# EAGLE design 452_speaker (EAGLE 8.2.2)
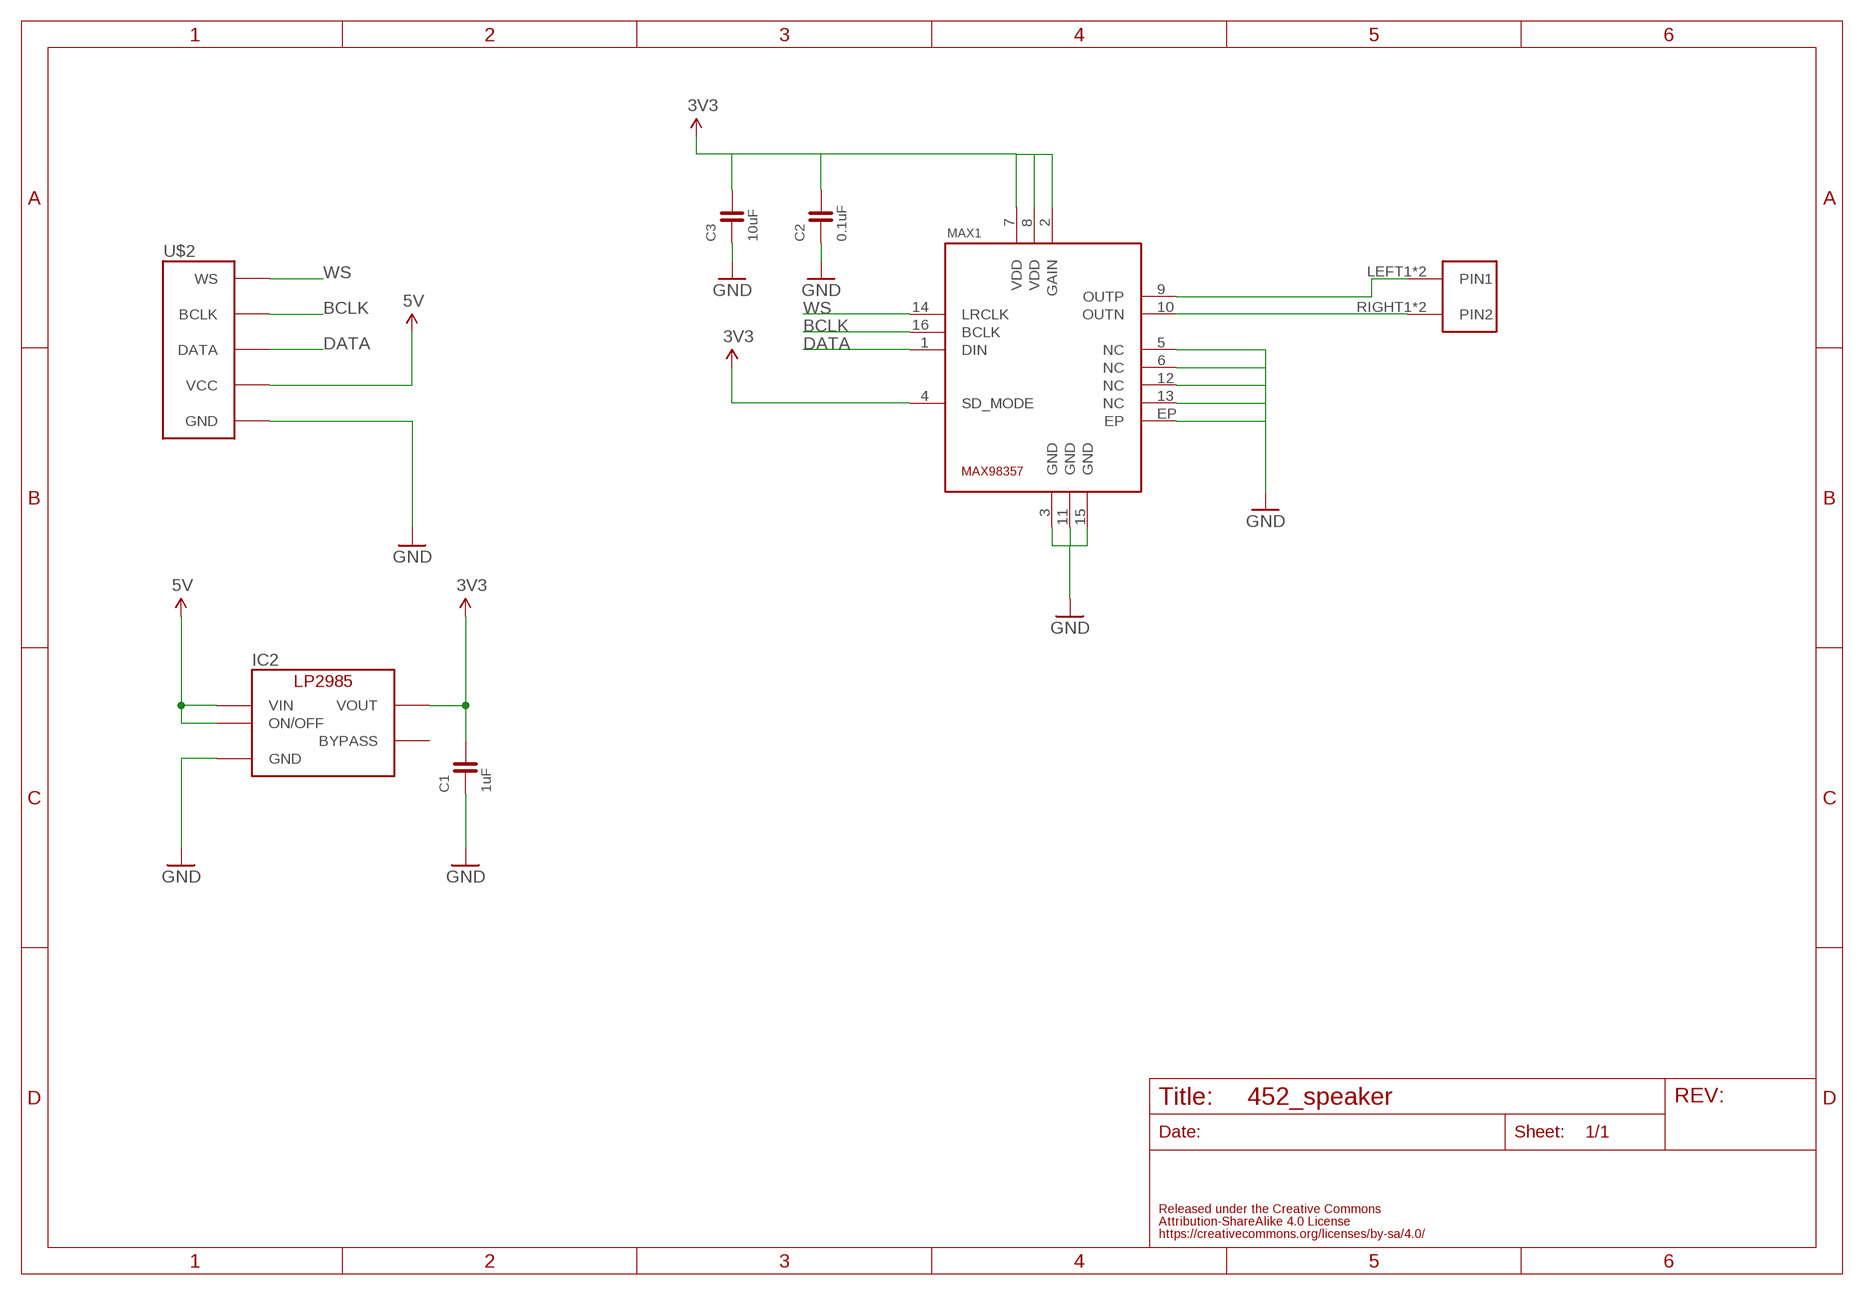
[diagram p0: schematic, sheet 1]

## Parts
C1  1uF  CAPACITOR-0603  [0603]
C2  0.1uF  CAPACITOR-0603  [0603]
C3  10uF  CAPACITOR-0603  [0603]
IC2  LP2985-33DBV  [SOT-23-5]
MAX1  MA-MAX98357  [MAXIM-MAX98357]
U$2  FABO_BRICK_I2S  [FABO_BRICK_I2S]
U$4  ML-1400-S1  [ML-1400-S1]

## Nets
3V3: C1.2 C2.2 C3.2 IC2.5(VOUT) MAX1.2(GAIN) MAX1.4(SD_MODE) MAX1.7(VDD) MAX1.8(VDD)
5V: IC2.1(VIN) IC2.3(ON/OFF) U$2.VCC
BCLK: MAX1.16(BCLK) U$2.BCLK
DATA: MAX1.1(DIN) U$2.DATA
GND: C1.1 C2.1 C3.1 IC2.2(GND) MAX1.3(GND) MAX1.5(NC) MAX1.6(NC) MAX1.11(GND) MAX1.12(NC) MAX1.13(NC) MAX1.15(GND) MAX1.EP U$2.GND
N$1: MAX1.10(OUTN) U$4.RIGHT1(PIN2) U$4.RIGHT2(PIN2)
N$2: MAX1.9(OUTP) U$4.LEFT1(PIN1) U$4.LEFT2(PIN1)
WS: MAX1.14(LRCLK) U$2.WS
Unconnected: IC2.4(BYPASS)

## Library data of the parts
C1-C3 = FaBo-Capacitor:CAPACITOR: CAPACITOR
IC2 = FaBo-Supply:LP2985: LP2985
MAX1 = FaBo-Mems:MA-MAX98357
U$2 = FaBo-Template:FABO_BRICK_I2S
U$4 = FaBo-Terminal:ML-1400-S1

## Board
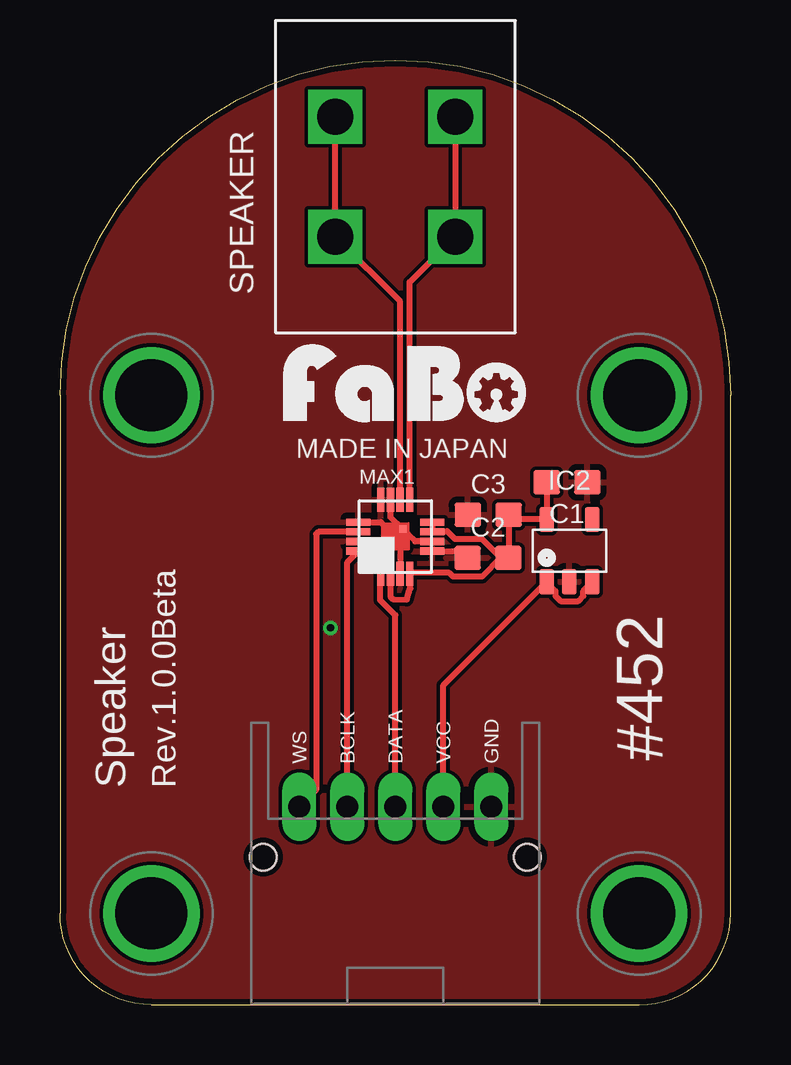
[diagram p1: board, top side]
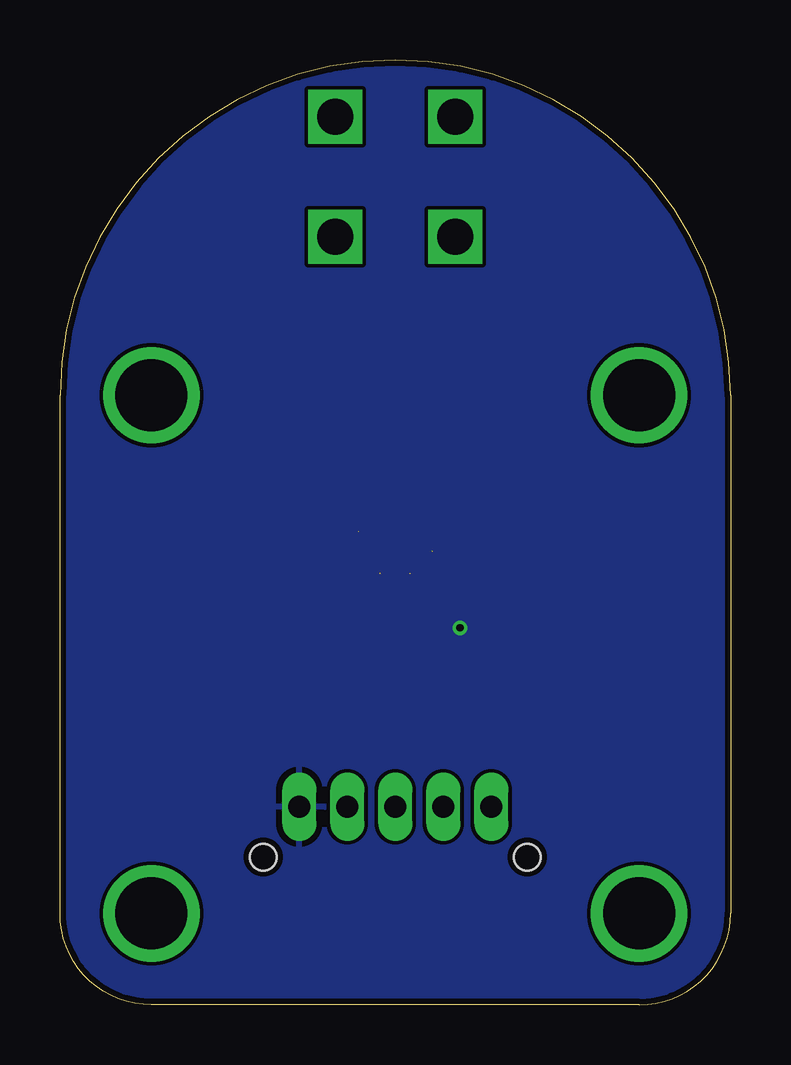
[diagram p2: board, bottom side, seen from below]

Size 27.94 x 39.37 mm. Coordinates in mm from the lower left corner, seen from the top.
Copper layers (1*16): Top 0.035mm / dielectric 1.5mm / Bottom 0.035mm
Design rules "Elecrow_angle": minimum track width 6mil, minimum drill 12mil, track to track 6mil, track to pad 6mil, pad to pad 6mil, via to via 6mil, smd to smd 0mil, copper to edge 10mil, drill to drill 10mil, minimum pad ring 10mil, minimum via ring 6mil, stop-mask expansion 2mil, vias tented up to drill 100mil, thermal gap 10mil

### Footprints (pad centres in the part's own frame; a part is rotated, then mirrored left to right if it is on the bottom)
0603 = smd 1.1 x 1: 1 -0.85,0; 2 0.85,0
SOT-23-5 = smd 0.6 x 1.05: 1 -0.95,-1.3; 2 0,-1.3; 3 0.95,-1.3; 4 0.95,1.3; 5 -0.95,1.3
MAXIM-MAX98357 = smd 0.3 x 1: 1 -0.6,-1.54; 2 -0.2,-1.54; 3 0.2,-1.54; 4 0.6,-1.54; 9 0.6,1.54; 10 0.2,1.54; 11 -0.2,1.54; 12 -0.6,1.54 | smd 1 x 0.3: 5 1.54,-0.6; 6 1.54,-0.2; 7 1.54,0.2; 8 1.54,0.6; 13 -1.54,0.6; 14 -1.54,0.2; 15 -1.54,-0.2; 16 -1.54,-0.6 | smd 0.3 x 0.3: EP 0.31,0.32
FABO_BRICK_I2S = drill 0.9 pad 1.422 long: BCLK -2,-8.255; DATA 0,-8.255; GND 4,-8.255; VCC 2,-8.255; WS -4,-8.255 | drill 3 pad 3.81: P$1 -10.16,8.89; P$2 10.16,8.89; P$3 -10.16,-12.7; P$4 10.16,-12.7 | hole 1.1: -5.5,-10.355; 5.5,-10.355
ML-1400-S1 = drill 1.5 square: LEFT1 -2.5,2.5; LEFT2 -2.5,-2.5; RIGHT1 2.5,2.5; RIGHT2 2.5,-2.5

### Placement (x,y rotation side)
C1  21.12,21.78 180 top
C2  17.84,18.62 0 top
C3  17.84,20.43 0 top
IC2  21.23,18.93 0 top
MAX1  13.97,19.51 0 top
U$2  13.97,16.51 0 top
U$3  [LOGO_FABO_MS]  14.37,23.91 0 top
U$4  13.97,34.51 180 top

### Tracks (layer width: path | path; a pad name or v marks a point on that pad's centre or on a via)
3V3  (3 unrouted)
  Top 0.254: C1.2 IC2.5 18.9,20.23 C3.2 18.7,18.64 C2.2 18.37,18.62 | 18.37,18.62 17.59,19.4 16.46,19.4 16.13,19.74 15.51,19.74 MAX1.8 | 18.37,18.62 17.59,17.85 16.38,17.85 16.22,18 14.6,18 | MAX1.2 13.77,17.01 13.87,16.91 14.45,16.89 14.54,17.19 14.6,17.35 14.6,17.97
5V
  Top 0.254: U$2.VCC 15.97,13.32 IC2.1 20.65,17.25 20.65,17.04 20.86,16.82 21.59,16.82 21.8,17.04 21.8,17.25 IC2.3
BCLK  (1 unrouted)
  Top 0.254: U$2.BCLK 11.97,18.45 12.4,18.88
DATA  (1 unrouted)
  Top 0.254: U$2.DATA 13.97,16.24 13.34,16.87 13.34,17.97
GND  (via drill 0.3)
  Top 0.254: MAX1.11 13.77,20.34 MAX1.EP 14.5,19.62 | MAX1.6 14.8,19.31 14.5,19.62 | MAX1.5 16.7,18.91 C2.1 | 14.17,19.29 MAX1.3 | 14.17,19.29 14.5,19.62 | MAX1.13 13.37,20.11 13.78,19.7 | 13.78,19.7 13.97,19.51 13.97,19.49 14.17,19.29 | MAX1.15 13.59,19.31 13.78,19.7
  other vias: 11.27,15.71 11.27,15.71
  pour Bottom: -0.03,-0.49 28.97,-0.49 28.97,39.51 -0.03,39.51
  pour Top: -0.03,-0.49 28.97,-0.49 28.97,39.51 -0.03,39.51
N$1
  Top 0.254: MAX1.10 14.17,29.31 U$4.RIGHT1 U$4.RIGHT2
N$2
  Top 0.254: MAX1.9 14.57,30.11 U$4.LEFT1 U$4.LEFT2
WS
  Top 0.254: MAX1.14 10.77,19.71 10.67,19.61 10.67,8.96 U$2.WS

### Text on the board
tPlace: SPEAKER | MADE IN JAPAN | #452 | Speaker | Rev.1.0.0Beta

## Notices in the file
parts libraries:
FaBo-etc: Released under the Creative Commons Attribution-ShareAlike 4.0 License
https://creativecommons.org/licenses/by-sa/4.0
FaBo-etc: Released under the Creative Commons
